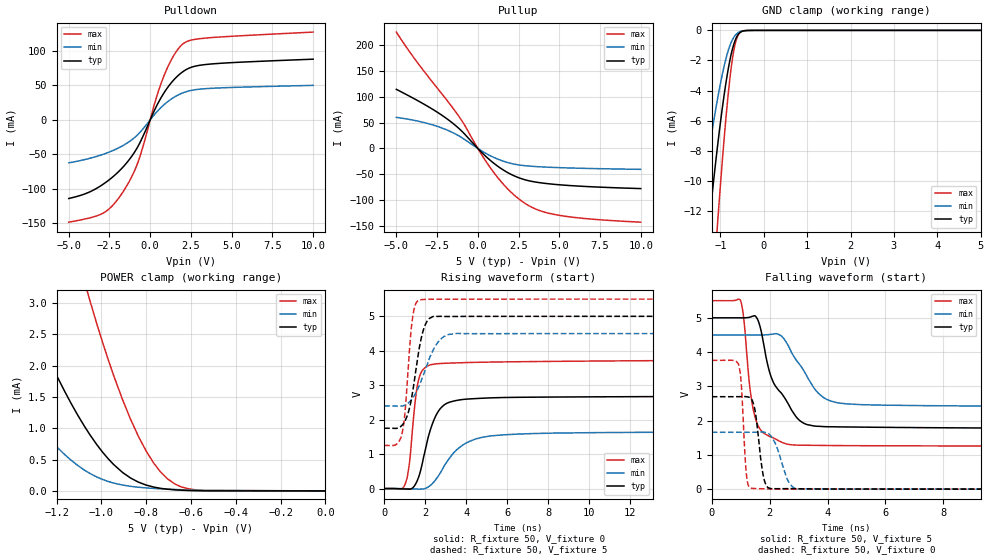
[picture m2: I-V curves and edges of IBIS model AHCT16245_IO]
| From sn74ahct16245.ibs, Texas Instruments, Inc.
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[Model]   AHCT16245_IO
Model_type  I/O
Vinl=0.8
Vinh=2.0
Enable   Active-Low
Vref =   0
Rref =   1000
Cref =   50p
Vmeas =   2.5
| variable   typ   min   max
C_comp   3.74pF   2.84pF   5.68pF
| C_pullup   4.30pF   2.88pF   5.68pF
| C_pulldown   3.80pF   3.01pF   4.99pF
| C_tri-state   3.13pF   2.84pF   3.58pF
[Temperature Range]   40   100   -40
| Ambient temperature   25   85   -40
[Voltage range]   5   4.5   5.5
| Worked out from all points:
|   slope of the pulldown table from 0 to 0.75 V, typ, clamps not added: 21.2 ohm
|   slope of the pullup table from 0 to 0.75 V, typ, clamps not added: 33.1 ohm
|   GND clamp passes 1 mA (typ) near -0.70 V on its own axis
|   POWER clamp passes 1 mA (typ) near -1.07 V on its own axis
|   rising waveform, R_fixture 50, V_fixture 0: 20-80 % time 767ps typ, 1.39ns min, 387ps max; typ from 0 V to 2.68 V
|   falling waveform, R_fixture 50, V_fixture 5: 20-80 % time 928ps typ, 953ps min, 352ps max; typ from 5 V to 1.76 V
|   rising waveform, R_fixture 50, V_fixture 5: 20-80 % time 543ps typ, 862ps min, 325ps max; typ from 1.75 V to 5 V
|   falling waveform, R_fixture 50, V_fixture 0: 20-80 % time 229ps typ, 389ps min, 142ps max; typ from 2.7 V to 0.001 V
[GND Clamp]
| AHCT16245_IO
|   Voltage   I(typ)   I(min)   I(max)
-5V       -171.6mA   -113.7mA   -217.6mA
-1.505V   -20.26mA   -12.83mA   -32.11mA
-1.275V   -13.24mA   -8.209mA   -21.63mA
-1.25V    -12.53mA   -7.741mA   -20.53mA
-1.075V   -7.895mA   -4.694mA   -13.2mA
-1.055V   -7.407mA   -4.375mA   -12.4mA
-880mV    -3.617mA   -1.963mA   -6.049mA
-770mV    -1.819mA   -923.1uA   -2.905mA
-670mV    -734.1uA   -369.7uA   -1.019mA
-620mV    -404uA     -214.5uA   -498.1uA
-550mV    -144.4uA   -89.73uA   -145.7uA
5V        60.98nA    4.363uA    569.7nA
[POWER Clamp]
| AHCT16245_IO
|   Voltage   I(typ)   I(min)   I(max)
-5V       72.18mA    45.57mA    118.1mA
-1.67V    6.352mA    3.259mA    13.63mA
-1.635V   5.949mA    3.021mA    12.9mA
-1.345V   3.016mA    1.333mA    7.407mA
-1.195V   1.81mA     689uA      5.004mA
-1.075V   1.029mA    331.2uA    3.34mA
-1.05V    891uA      277.3uA    3.026mA
-870mV    207uA      73.47uA    1.148mA
-800mV    93.38uA    48.11uA    636.5uA
-705mV    27.52uA    28.58uA    193.4uA
-580mV    3.207uA    11.82uA    17.38uA
-84.45fV  60.98nA    3.404nA    872.2nA
[Pulldown]
| AHCT16245_IO
|   Voltage   I(typ)   I(min)   I(max)
-5V       -114mA     -62.37mA   -148.4mA
-3.835V   -105.7mA   -56.56mA   -142.8mA
-2.85V    -92.69mA   -49.65mA   -134.7mA
-2.275V   -82.24mA   -44.36mA   -123.3mA
-1.62V    -67.18mA   -36.57mA   -102.6mA
-710mV    -36.71mA   -20.21mA   -58.75mA
335mV     17.41mA    9.686mA    28.84mA
855mV     39.41mA    22.04mA    64.38mA
1.45V     57.97mA    32.5mA     93.4mA
2.015V    69.91mA    39.15mA    110.2mA
3.58V     80.57mA    45.43mA    118.8mA
10V       87.89mA    49.93mA    127.1mA
[Pullup]
| AHCT16245_IO
|   Voltage   I(typ)   I(min)   I(max)
-5V       114.2mA    60mA       224.9mA
-3.725V   92.97mA    53.13mA    166.8mA
-1.74V    53.65mA    33.49mA    86.72mA
-925mV    31.52mA    19.65mA    50.78mA
135mV     -4.451mA   -2.78mA    -7.049mA
895mV     -26.47mA   -16.08mA   -42.9mA
1.71V     -44.45mA   -26.08mA   -74.12mA
2.525V    -56.78mA   -31.93mA   -97.85mA
3.535V    -64.91mA   -34.96mA   -116.9mA
4.77V     -69.59mA   -36.84mA   -128mA
6.78V     -73.77mA   -38.65mA   -136mA
10V       -77.6mA    -40.43mA   -142.5mA
[Ramp]
| AHCT16245_IO
| variable   typ   min   max
dV/dt_r   1.62/7.89E-10   1.00/1.45E-09   2.25/3.98E-10
dV/dt_f   1.98/9.29E-10   1.28/9.86E-10   2.58/3.57E-10
R_load = 50
[Rising Waveform]
| AHCT16245_IO
R_fixture =   50
C_fixture =   0
L_fixture =   0
V_fixture =   0
V_fixture_min = 0
V_fixture_max = 0
|   Time   V(typ)   V(min)   V(max)
0s        7.005uV    -5.289uV   14.22uV
1.03ns    -12.95mV   -3.869mV   141.7mV
1.245ns   -17.23mV   -7.113mV   799.4mV
1.485ns   86.25mV    -10.99mV   2.377V
1.65ns    284.7mV    -15.43mV   3.08V
2.29ns    1.775V     111mV      3.595V
3.065ns   2.478V     783mV      3.638V
3.96ns    2.593V     1.31V      3.655V
5.24ns    2.633V     1.531V     3.671V
24.99ns   2.684V     1.65V      3.737V
[Falling Waveform]
| AHCT16245_IO
R_fixture =   50
C_fixture =   0
L_fixture =   0
V_fixture =   5
V_fixture_min = 4.5
V_fixture_max = 5.5
|   Time   V(typ)   V(min)   V(max)
0s        5V         4.5V       5.5V
985ps     5V         4.5V       5.523V
1.11ns    4.998V     4.5V       4.941V
1.34ns    5.025V     4.5V       2.807V
1.535ns   5.023V     4.499V     1.995V
2.055ns   3.267V     4.518V     1.522V
2.635ns   2.5V       4.199V     1.31V
3.685ns   1.834V     2.799V     1.278V
4.645ns   1.815V     2.49V      1.271V
24.99ns   1.758V     2.404V     1.253V
[Rising Waveform]
| AHCT16245_IO
R_fixture =   50
C_fixture =   0
L_fixture =   0
V_fixture =   5
V_fixture_min = 4.5
V_fixture_max = 5.5
|   Time   V(typ)   V(min)   V(max)
0s        1.751V     2.4V       1.252V
855ps     1.827V     2.396V     1.551V
1.015ns   1.964V     2.423V     2.208V
1.365ns   2.725V     2.607V     4.868V
1.515ns   3.314V     2.746V     5.324V
1.71ns    4.073V     2.989V     5.47V
2.185ns   4.928V     3.741V     5.493V
2.735ns   4.998V     4.324V     5.496V
3.45ns    4.995V     4.498V     5.497V
24.99ns   5V         4.5V       5.5V
[Falling Waveform]
| AHCT16245_IO
R_fixture =   50
C_fixture =   0
L_fixture =   0
V_fixture =   0
V_fixture_min = 0
V_fixture_max = 0
|   Time   V(typ)   V(min)   V(max)
0s        2.698V     1.66V      3.759V
920ps     2.699V     1.66V      3.651V
1.02ns    2.701V     1.66V      3.05V
1.2ns     2.698V     1.66V      416.4mV
1.385ns   2.611V     1.66V      25.61mV
1.785ns   371.4mV    1.666V     12.27mV
2.035ns   17.09mV    1.558V     8.721mV
2.645ns   15.85mV    229.8mV    6.221mV
3.02ns    11.79mV    8.981mV    3.815mV
24.99ns   532.1uV    617.3uV    406.6uV
